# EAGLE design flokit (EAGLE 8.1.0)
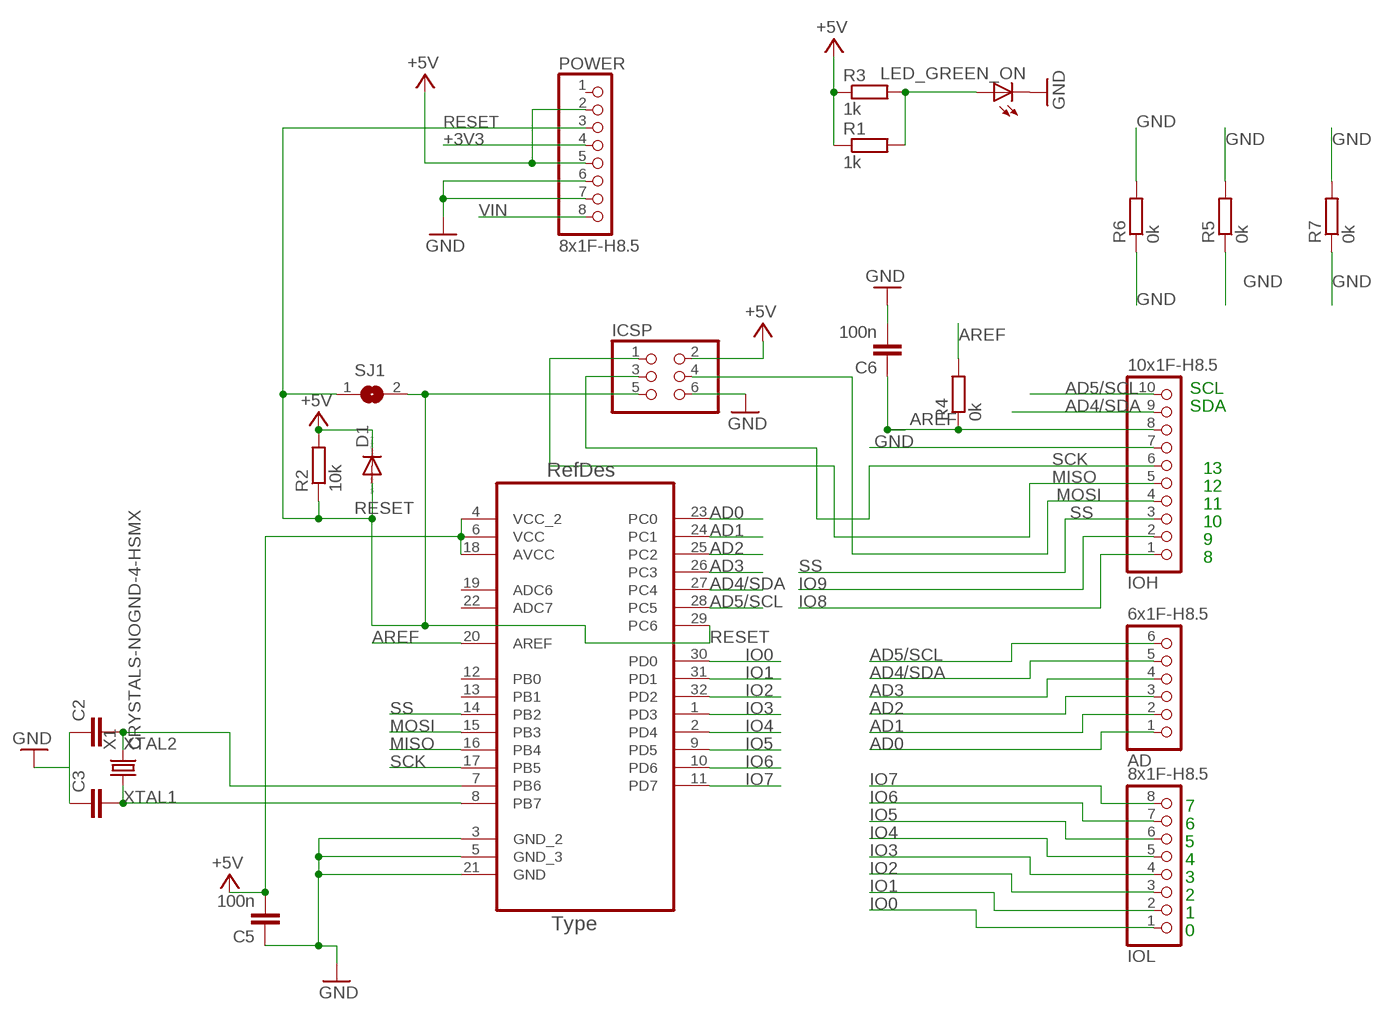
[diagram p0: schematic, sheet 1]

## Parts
AD  6x1F-H8.5  PINHD-1X6  [1X06]
ATMEGA328P  ATMEGA328P-AU  [QFP80P900X900X120-32N]
C2  C-EUC0603K  [C0603K]
C3  C-EUC0603K  [C0603K]
C5  100n  C-EUC0603K  [C0603K]
C6  100n  C-EUC0603K  [C0603K]
D1  DIODE-DO214AC  [DO214AC]
ICSP  PINHD-2X3SMT  [2X03_SMT]
IOH  10x1F-H8.5  PINHD-1X10_ARD  [1X10]
IOL  8x1F-H8.5  PINHD-1X8  [1X08]
LED_GREEN_ON  LEDCHIPLED_1206  [CHIPLED_1206]
POWER  8x1F-H8.5  PINHD-1X8  [1X08]
R1  1k  R-EU_M1206  [M1206]
R2  10k  R-EU_M1206  [M1206]
R3  1k  R-EU_M1206  [M1206]
R4  0k  R-EU_M1206  [M1206]
R5  0k  R-EU_M1206  [M1206]
R6  0k  R-EU_M1206  [M1206]
R7  0k  R-EU_M1206  [M1206]
SJ1  SJW  [SJW]
X1  CRYSTALS-NOGND-4-HSMX  [HC49-4-HSMX]

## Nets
+3V3: POWER.4
+5V [usbvcc]: ATMEGA328P.4(VCC_2) ATMEGA328P.6(VCC) ATMEGA328P.18(AVCC) C5.2 D1.C ICSP.2 POWER.2 POWER.5 R1.1 R2.2 R3.1
AD0: AD.1 ATMEGA328P.23(PC0)
AD1: AD.2 ATMEGA328P.24(PC1)
AD2: AD.3 ATMEGA328P.25(PC2)
AD3: AD.4 ATMEGA328P.26(PC3)
AD4/SDA: AD.5 ATMEGA328P.27(PC4) IOH.9
AD5/SCL: AD.6 ATMEGA328P.28(PC5) IOH.10
AREF [aref]: ATMEGA328P.20(AREF) C6.1 IOH.8 R4.1 R4.2
GND [gnd]: ATMEGA328P.3(GND_2) ATMEGA328P.5(GND_3) ATMEGA328P.21(GND) C2.1 C3.1 C5.1 C6.2 ICSP.6 IOH.7 LED_GREEN_ON.C POWER.6 POWER.7 R5.1 R5.2 R6.1 R6.2 R7.1 R7.2
IO0: ATMEGA328P.30(PD0) IOL.1
IO1: ATMEGA328P.31(PD1) IOL.2
IO2: ATMEGA328P.32(PD2) IOL.3
IO3: ATMEGA328P.1(PD3) IOL.4
IO4: ATMEGA328P.2(PD4) IOL.5
IO5: ATMEGA328P.9(PD5) IOL.6
IO6: ATMEGA328P.10(PD6) IOL.7
IO7: ATMEGA328P.11(PD7) IOL.8
IO8: IOH.1
IO9: IOH.2
MISO: ATMEGA328P.16(PB4) ICSP.1 IOH.5
MOSI: ATMEGA328P.15(PB3) ICSP.4 IOH.4
N$3: LED_GREEN_ON.A R1.2 R3.2
RESET: ATMEGA328P.29(PC6) D1.A ICSP.5 POWER.3 R2.1 SJ1.1 SJ1.2
SCK: ATMEGA328P.17(PB5) ICSP.3 IOH.6
SS: ATMEGA328P.14(PB2) IOH.3
VIN [power]: POWER.8
XTAL1: ATMEGA328P.8(PB7) C3.2 X1.1
XTAL2: ATMEGA328P.7(PB6) C2.2 X1.2
Unconnected: ATMEGA328P.12(PB0) ATMEGA328P.13(PB1) ATMEGA328P.19(ADC6) ATMEGA328P.22(ADC7) POWER.1

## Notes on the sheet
- SCL
- SDA
- 13
- 12
- 11
- 10
- 9
- 8
- 7
- 6
- 5
- 4
- 3
- 2
- 1
- 0

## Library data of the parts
AD = SmartPrj:PINHD-1X6: PIN HEADER
ATMEGA328P = Atmel-ATMEGA328P-AU:ATMEGA328P-AU; DESCRIPTION: 8-bit Microcontroller with In-System Programmable Flash; MPN: ATMEGA328P-AU; OC_FARNELL: 1715486; OC_NEWARK: 14R4631; PACKAGE: TQFP-32; SUPPLIER: Atmel
C2 C3 C5 C6 = resistor:C-EU: CAPACITOR, European symbol
D1 = diode:DIODE-: DIODE
ICSP = pinhead+:PINHD-2X3: PIN HEADER
IOH = SmartPrj:PINHD-1X10_ARD: PIN HEADER
IOL POWER = SmartPrj:PINHD-1X8: PIN HEADER
LED_GREEN_ON = led:LED: LED
R1-R7 = resistor:R-EU_: RESISTOR, European symbol
SJ1 = jumper:SJ: SMD solder JUMPER
X1 = IQD-Frequency-Products:CRYSTALS-NOGND: CRYSTALS CAN NOT GROUNDED

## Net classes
0 default: width 0.254 mm, clearance 0.254 mm
1 power: width 0.61 mm, drill 0.61 mm, clearance 0.254 mm
2 gnd: width 0.305 mm, drill 0.559 mm, clearance 0.254 mm
3 usbvcc: width 0.508 mm, drill 0.61 mm, clearance 0.254 mm
4 aref: width 0.406 mm, drill 0.61 mm, clearance 0.254 mm

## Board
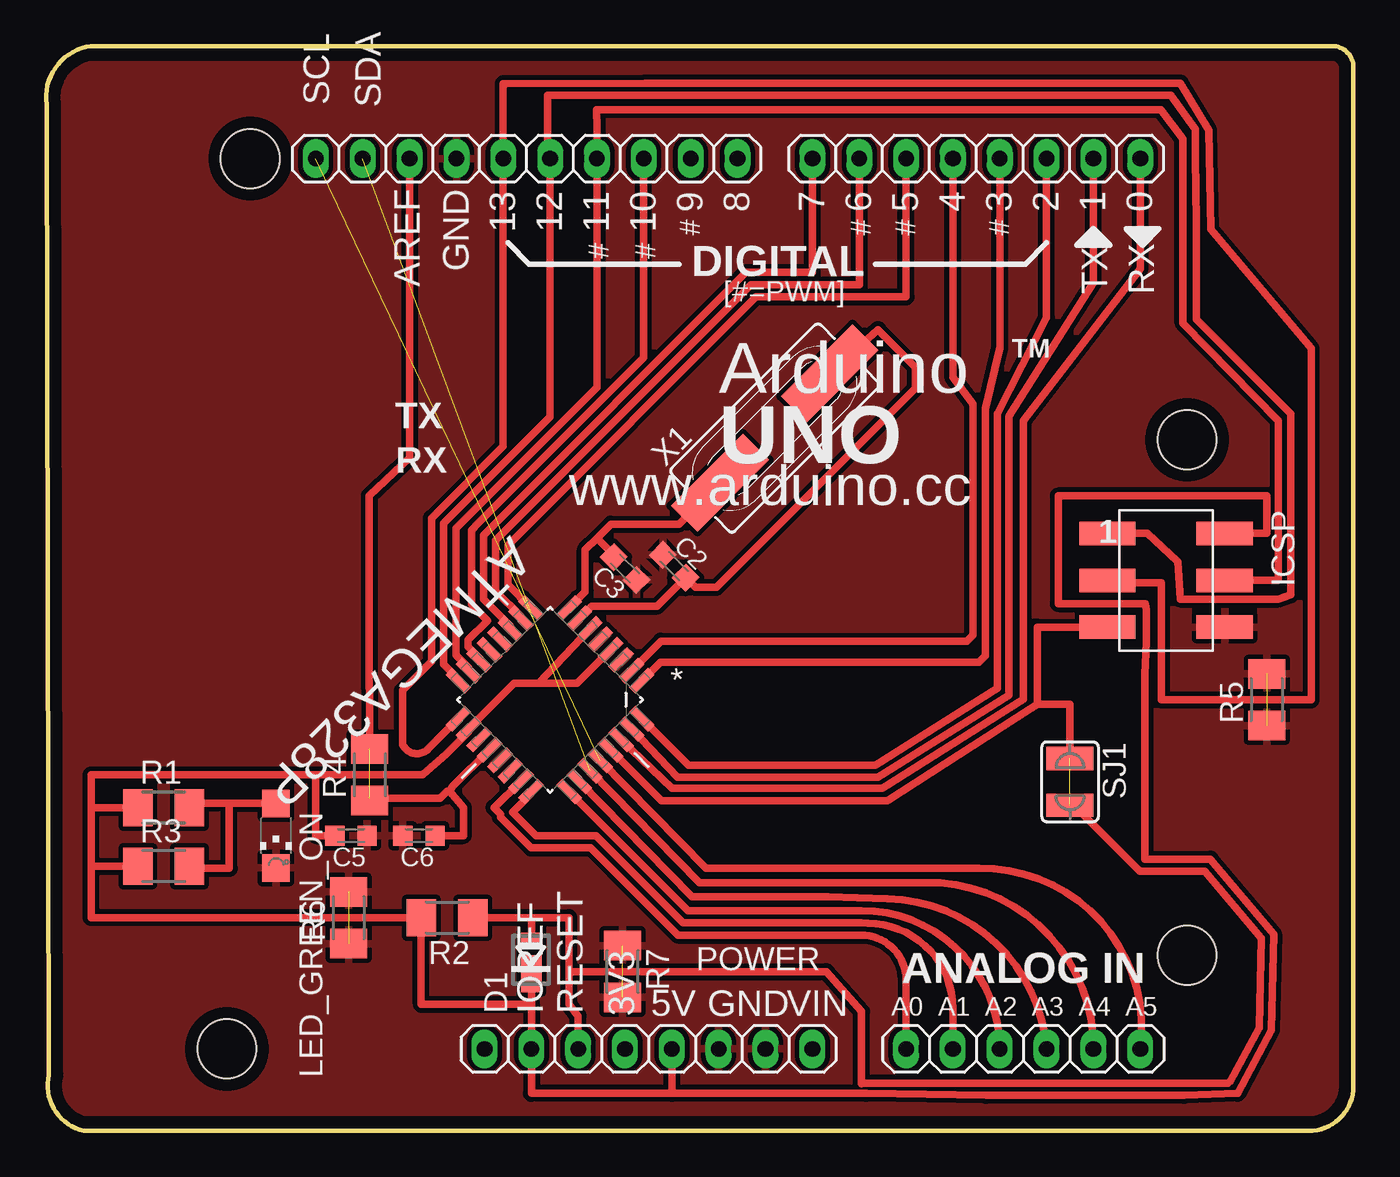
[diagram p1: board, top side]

Size 70.89 x 58.8 mm. Coordinates in mm from the lower left corner, seen from the top.
Outline: 70.89,57.66 70.89,2.41 arc-90 68.48,0 2.04,0 arc-90 0.15,3.03 0.02,55.64 arc-90 2.42,58.8 69.75,58.8 arc-90 70.89,57.66
Copper layers (1*16): Top 0.035mm / dielectric 1.5mm / Bottom 0.035mm
Design rules "default": minimum track width 10mil, minimum drill 22mil, track to track 10mil, track to pad 10mil, pad to pad 10mil, via to via 12mil, smd to smd 8mil, copper to edge 26mil, drill to drill 12mil, minimum pad ring 10mil, minimum via ring 10mil, stop-mask expansion 1mil, vias tented up to drill 30mil, thermal gap 10mil
Holes 3.2 mm at 61.87,37.47 61.87,9.53 11.07,52.7 9.8,4.45
vRestrict: area 18.7,46 to 20.5,51.1; area 21.2,47.4 to 22.9,51.1; area 24.3,47.2 to 25.4,50.7; area 26.8,47.2 to 28,50.7; area 29.4,47.2 to 30.5,50.7; area 31.9,47.2 to 33,50.7; area 34.6,49.1 to 35.7,50.7; area 36.1,47 to 43.5,48.8; area 56.2,46.1 to 57.6,48.6; area 58.7,46.1 to 60.1,48.6; area 57.2,37.7 to 60.6,39.1; area -3.5,23.7 to -2.1,32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

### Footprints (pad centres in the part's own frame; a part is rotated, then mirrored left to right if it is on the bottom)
1X06 = drill 0.85 pad 1.422 long: 1 -6.35,0; 2 -3.81,0; 3 -1.27,0; 4 1.27,0; 5 3.81,0; 6 6.35,0
QFP80P900X900X120-32N = smd 1.473 x 0.508: 1 -4.242,2.794; 2 -4.242,2.007; 3 -4.242,1.194; 4 -4.242,0.406; 5 -4.242,-0.406; 6 -4.242,-1.194; 7 -4.242,-2.007; 8 -4.242,-2.794; 17 4.242,-2.794; 18 4.242,-2.007; 19 4.242,-1.194; 20 4.242,-0.406; 21 4.242,0.406; 22 4.242,1.194; 23 4.242,2.007; 24 4.242,2.794 | smd 0.508 x 1.473: 9 -2.794,-4.242; 10 -2.007,-4.242; 11 -1.194,-4.242; 12 -0.406,-4.242; 13 0.406,-4.242; 14 1.194,-4.242; 15 2.007,-4.242; 16 2.794,-4.242; 25 2.794,4.242; 26 2.007,4.242; 27 1.194,4.242; 28 0.406,4.242; 29 -0.406,4.242; 30 -1.194,4.242; 31 -2.007,4.242; 32 -2.794,4.242
C0603K = smd 1.05 x 1.08: 1 -0.875,0; 2 0.875,0
DO214AC = smd 0.813 x 1.092: A 1.321,0 | smd 2.007 x 1.092: C -0.508,0
2X03_SMT = smd 1.27 x 3.048: 1 -2.54,-3.175; 2 -2.54,3.175; 3 0,-3.175; 4 0,3.175; 5 2.54,-3.175; 6 2.54,3.175
1X10 = drill 0.85 pad 1.422 long: 1 -11.43,0; 2 -8.89,0; 3 -6.35,0; 4 -3.81,0; 5 -1.27,0; 6 1.27,0; 7 3.81,0; 8 6.35,0; 9 8.89,0; 10 11.43,0
1X08 = drill 0.85 pad 1.422 long: 1 -8.89,0; 2 -6.35,0; 3 -3.81,0; 4 -1.27,0; 5 1.27,0; 6 3.81,0; 7 6.35,0; 8 8.89,0
CHIPLED_1206 = smd 1.5 x 1.5: A 0,-1.75; C 0,1.75
M1206 = smd 1.6 x 2: 1 -1.4,0; 2 1.4,0
SJW = smd 1.27 x 2.54: 1 -1.27,0; 2 1.27,0
HC49-4-HSMX = smd 5.5 x 2: 1 -4.2,0; 2 4.2,0

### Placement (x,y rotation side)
AD  52.98,4.45 0 top
ATMEGA328P  27.33,23.37 225 top
C2  34.06,30.61 315 top
C3  31.39,30.48 135 top
C5  16.53,16 180 top
C6  20.22,16 180 top
D1  26.31,9.02 90 top
ICSP  60.73,29.85 270 top
IOH  26.06,52.7 180 top
IOL  50.44,52.7 180 top
LED_GREEN_ON  12.47,16 180 top
POWER  32.66,4.45 0 top
R1  6.37,17.53 0 top
R2  21.74,11.56 180 top
R3  6.37,14.35 0 top
R4  17.55,19.3 90 top
R5  66.19,23.37 90 top
R6  16.41,11.56 90 top
R7  31.27,8.64 270 top
SJ1  55.52,18.92 270 top
X1  39.52,38.1 45 top

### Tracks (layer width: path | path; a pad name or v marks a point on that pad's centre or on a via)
+5V
  Top 0.406: ATMEGA328P.6 26.69,24.26 | 26.69,24.26 25.38,24.26 ATMEGA328P.18 22.91,21.64 21.69,20.42 20.43,19.3 14.63,19.3 | 26.69,24.26 28.79,24.26 ATMEGA328P.4 | 26.31,6.86 D1.C | 33.93,2.03 POWER.5 | 33.93,2.03 26.31,2.03 POWER.2 26.31,6.86 | ICSP.2 66.19,32.38 66.19,34.42 54.89,34.42 54.89,28.58 59.6,28.58 59.66,28.26 59.66,26.48 59.59,24.75 59.59,14.73 63.14,14.73 66.57,10.67 66.44,5.46 64.62,2.03 61.72,1.93 50.98,1.93 44.47,2.03 33.93,2.03 | 26.31,6.86 20.34,6.86 R2.2 2.44,11.56 2.44,14.35 | R1.1 2.44,17.53 | 2.44,14.35 2.44,17.53 | 2.44,14.35 R3.1 | 2.44,17.53 2.44,19.3 14.63,19.3 | 14.63,19.3 14.63,16 C5.2
AD0
  Top 0.406: ATMEGA328P.23 24.28,17.53 24.64,17.17 24.64,17 26.29,15.34 29.54,15.34 34.26,10.62 44.19,10.62 arc-90 46.63,8.17 AD.1
AD1
  Top 0.406: ATMEGA328P.24 26.3,18.28 25.3,17.27 26.57,16 29.81,16 34.53,11.28 44.22,11.28 44.56,11.25 arc-90 49.17,6.64 AD.2
AD2
  Top 0.406: ATMEGA328P.25 34.81,11.94 44.22,11.94 arc-90 AD.3
AD3
  Top 0.406: ATMEGA328P.26 35.03,12.7 40.79,12.7 arc-3 45.62,12.57 arc-84 AD.4
AD4/SDA  (1 unrouted)
  Top 0.406: ATMEGA328P.27 35.42,13.46 47.65,13.46 arc-92 AD.5
AD5/SCL  (1 unrouted)
  Top 0.406: ATMEGA328P.28 35.77,14.22 50.57,14.22 arc-99 AD.6
AREF  (1 unrouted)
  Top 0.406: C6.1 22.63,16 22.63,17.53 21.87,18.42 | 21.87,18.42 22.05,18.67 ATMEGA328P.20 | IOH.8 19.71,36.49 17.52,34.44 17.52,25.5 17.55,22.35 R4.2 | 21.87,18.42 21.74,18.41 21.36,18.03 17.55,18.03 R4.1
GND  (3 unrouted)
  pour Top: -6.58,59.94 71.4,59.56 71.4,-2.79 -6.83,-2.41
IO0
  Top 0.406: ATMEGA328P.30 33.94,18.57 45.36,18.57 52.98,23.39 52.98,38.48 59.33,46.74 IOL.1
IO1
  Top 0.406: ATMEGA328P.31 34.23,19.18 45.11,19.18 52.22,23.62 52.22,38.73 56.79,45.97 IOL.2
IO2
  Top 0.406: ATMEGA328P.32 34.84,19.81 44.98,19.81 51.59,24 51.59,38.86 54.25,44.07 IOL.3
IO3
  Top 0.406: ATMEGA328P.1 33.31,25.4 50.57,25.4 50.93,25.76 50.93,39.14 51.71,42.46 IOL.4
IO4
  Top 0.406: ATMEGA328P.2 33.34,26.54 49.93,26.54 50.26,26.87 50.26,39.41 49.17,40.86 IOL.5
IO5
  Top 0.406: ATMEGA328P.9 25.04,29.61 25.04,31.75 38.5,45.21 46.63,45.21 IOL.6
IO6
  Top 0.406: ATMEGA328P.10 25.75,27.89 24.38,29.26 24.38,32.02 38.23,45.87 44.09,45.87 IOL.7
IO7
  Top 0.406: ATMEGA328P.11 25.17,27.36 23.72,28.81 23.72,32.3 37.96,46.53 38.5,46.53 | 38.5,46.53 | 38.5,46.53 41.55,46.53 IOL.8
MISO
  Top 0.406: ATMEGA328P.16 22.35,24.5 21.56,25.29 21.56,32.94 27.33,38.71 IOH.5 27.2,52.83 27.2,56.13 60.98,56.13 62.3,54.3 62.3,52.78 62.38,49.28 62.38,43.99 67.49,38.88 67.49,29.06 66.83,28.83 61.49,28.83 61.36,30.86 59.71,32.38 ICSP.1
MOSI
  Top 0.406: ATMEGA328P.15 22.91,25.09 22.22,25.78 22.22,32.67 29.87,40.31 IOH.4 29.87,54.36 29.84,55.35 60.45,55.35 61.64,53.77 61.64,43.79 66.83,38.48 66.83,29.85 ICSP.4
N$3
  Top 0.406: R1.2 7.77,17.75 10.18,17.75 | 10.18,17.75 LED_GREEN_ON.A | R3.2 7.77,14.22 9.93,14.22 9.93,17.75 10.18,17.75
RESET  (1 unrouted)
  Top 0.406: ATMEGA328P.29 33.36,17.91 45.62,17.91 53.74,23.11 | 53.74,23.11 53.74,27.3 ICSP.5 | 26.31,11.56 R2.1 | 26.31,11.56 28.34,11.56 28.34,8.5 | 28.34,8.38 28.34,8.5 | 58.93,14.46 58.93,14.45 | 59.32,14.07 59.31,14.07 58.93,14.46 | 59.32,14.07 | 28.48,8.63 42.31,8.64 44.22,6.48 44.22,2.56 44.22,2.57 47.51,2.59 58.91,2.59 60.69,2.59 61.34,2.59 61.61,2.59 62,2.59 64.08,2.57 64.2,2.7 65.78,5.6 65.81,6.86 65.82,6.86 65.91,10.43 62.84,14.07 59.32,14.07 | 28.48,8.63 28.34,8.38 | D1.A 26.31,11.56 | POWER.3 28.85,6.22 28.34,6.86 28.34,8.38 | 28.34,8.5 28.48,8.63 | 53.74,23.11 55.52,23.11 SJ1.1 | SJ1.2 55.73,17.65 58.93,14.46
SCK
  Top 0.406: ATMEGA328P.17 22.35,22.33 20.72,20.7 arc-111 19.33,20.96 19.33,23.88 20.9,25.45 20.9,33.21 24.79,37.1 IOH.6 24.79,56.77 24.95,56.77 32.47,56.79 61.51,56.79 63.04,54.24 63.17,48.87 68.6,42.42 68.6,23.37 60.48,23.37 60.48,29.72 57.68,29.72 ICSP.3
SS
  Top 0.406: ATMEGA328P.14 23.52,25.59 22.88,26.23 22.88,26.61 23.93,27.66 23.06,28.53 23.06,32.57 23.45,32.96 | 23.45,32.96 | IOH.3 32.41,41.92 23.45,32.96
XTAL1
  Top 0.406: C3.2 30.77,31.23 29.87,32.13 | 29.87,32.13 30.63,32.89 34.31,32.89 X1.1 36.8,35.38 | ATMEGA328P.8 29.23,29.22 29.23,31.5 29.87,32.13
XTAL2
  Top 0.406: ATMEGA328P.7 29.57,28.45 33.14,28.45 C2.2 35.2,29.46 36.35,29.46 47.14,40.26 47.14,41.4 45.11,43.43 X1.2

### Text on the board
tPlace: 13 | 12 | 11 | 10 | 9 | 8 | 7 | 6 | 5 | 4 | 3 | 2 | 1 | 0
tNames: SCL | SDA | M.Banzi | D.Cuartielles | T.Igoe | AREF | GND | G.Martino | # | # | # | # | D.Mellis | # | # | DIGITAL | [#=PWM] | TX | RX | TM | TX | Arduino | RX | UNO | www.arduino.cc | 1 | ANALOG IN | IOREF | RESET | 3V3 | 5V | GND | VIN | A0 | A1 | A2 | A3 | A4 | A5
bNames: MADE IN | designed by | MADE IN | ITALY | tinker it | ITALY | designed by | tinker it | ATMEGA328
ReferenceLC: L | TX | ON | RX | PC1 | PC2
214bmp: D:/SmartProjects/Snc/a4_bn_logo2.bmp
